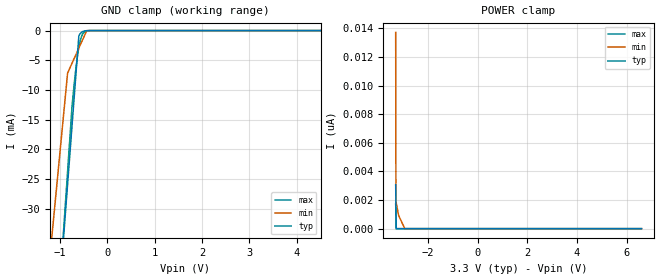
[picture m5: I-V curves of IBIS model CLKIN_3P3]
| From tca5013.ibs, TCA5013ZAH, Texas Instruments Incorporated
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[Model]   CLKIN_3P3
Model_type   Input
Vinl = .66
Vinh = 2.64
|   typ   min   max
C_comp   0.731p   0.503p   0.930p
[Model spec]
|subparameter
Vinl   0.66   0.6   0.72
Vinh   2.64   2.4   2.88
[Voltage Range]   3.3   3   3.6
[Temperature Range]   27   125   -40
[Power Clamp Reference]   3.3   3   3.6
[GND Clamp Reference]   0   0   0
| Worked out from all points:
|   GND clamp passes 1 mA (typ) near -0.60 V on its own axis
[GND Clamp]
|   Voltage   I(typ)   I(min)   I(max)
-3.3V     -708.9mA   -336.7mA   -997mA
-1.191V   -63.43mA   -36.72mA   -65.44mA
-834.9mV  -25.88mA   -7.155mA   -23.73mA
-735.9mV  -15.45mA   -5.401mA   -12.32mA
-666.6mV  -8.15mA    -4.174mA   -6.818mA
-627mV    -3.978mA   -3.473mA   -4.316mA
-597.9mV  -913.4uA   -2.957mA   -2.856mA
-557.7mV  -411.8uA   -2.245mA   -1.411mA
-508.2mV  -134.5uA   -1.368mA   -472.5uA
-432.1mV  -19.06uA   -20.48uA   -58.91uA
-389.4mV  -5.567uA   -7.609uA   -14.63uA
6.6V      0A         0A         0A
[POWER Clamp]
|   Voltage   I(typ)   I(min)   I(max)
-3.3V     3.076nA    13.73nA    1.738nA
-3.29V    1.538nA    1.921nA    869.2pA
-3.28V    0A         1.826nA    0A
-3.181V   0A         919.2pA    0A
-2.934V   0A         0A         0A
6.6V      0A         0A         0A
